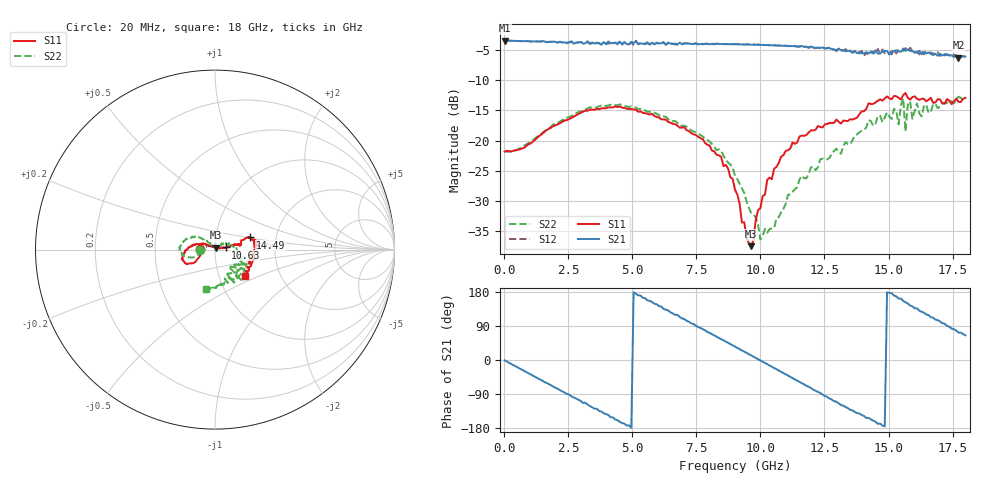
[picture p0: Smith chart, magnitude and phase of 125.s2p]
!Agilent Technologies,N5230A,US43500223,A.07.50.48
!Agilent N5230A: A.07.50.48
!Date: Monday, January 11, 2016 21:20:18
!Correction: S11(Full 2 Port(1,2))
!S21(Full 2 Port(1,2))
!S12(Full 2 Port(1,2))
!S22(Full 2 Port(1,2))
!S2P File: Measurements: S11, S21, S12, S22:
# Hz S  dB  R 50
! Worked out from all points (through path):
!   201 points, 20 MHz to 18 GHz, reference 50 ohm
!   highest |S21| = -3.44 dB at 20 MHz (marker M1); lowest = -6.3 dB at 17.73 GHz (marker M2)
!   group delay of S21, straight-line fit = 101 ps
!   lowest |S11| = -37.5 dB at 9.639 GHz (marker M3), VSWR 1.03, Z = 50.7 + j1.15 ohm
!   |S11| at or under -10 dB: start of sweep to end of sweep
!   |S22| runs from -36.4 to -12.7 dB; largest |S21 - S12| = 0.057
!   S11 on the Smith chart (normalised r, x): 20 MHz: 0.85, +0.00; 10.63 GHz: 1.13, +0.03; 14.49 GHz: 1.47, +0.21; 18 GHz: 1.33, -0.42
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2e7  -21.83 179.4  -3.44 -0.9  -3.43 -0.9  -21.76 180.0
1.5483e9  -18.66 -150.3  -3.54 -57.0  -3.57 -56.9  -18.55 -159.5
3.0766e9  -15.21 -153.1  -3.95 -113.3  -3.80 -112.2  -15.12 -168.7
4.515e9  -14.35 -165.2  -3.63 -163.2  -3.48 -162.3  -14.02 176.0
6.0433e9  -16.17 179.2  -3.92 142.1  -3.93 141.6  -15.78 157.3
7.4817e9  -19.07 163.7  -3.87 90.6  -4.00 90.9  -18.63 143.6
9.01e9  -28.14 149.7  -4.07 35.3  -4.02 35.6  -25.82 132.0
9.6393e9  -37.47 57.9  -4.14 12.2  -4.12 12.5  -31.96 114.4
9.9989e9  -31.19 10.7  -4.15 -1.3  -4.17 -0.8  -36.38 96.3
1.06282e10  -24.37 11.7  -4.28 -24.1  -4.25 -24.2  -32.86 51.4
1.20666e10  -18.33 13.7  -4.62 -78.4  -4.57 -77.7  -24.30 35.5
1.33252e10  -16.73 12.2  -5.22 -124.1  -4.85 -124.0  -20.26 14.3
1.44939e10  -13.71 19.2  -5.07 -163.0  -5.60 -159.7  -17.20 -13.3
1.50333e10  -13.02 12.5  -5.78 177.0  -5.43 175.9  -16.02 -33.4
1.53929e10  -12.94 8.2  -5.23 162.2  -5.00 167.0  -17.32 -38.4
1.55727e10  -12.49 5.4  -4.78 156.0  -5.18 161.2  -13.00 -49.1
1.56626e10  -12.12 5.0  -5.15 152.3  -4.68 153.2  -18.46 -51.1
1.58424e10  -13.22 4.3  -5.15 143.7  -4.63 145.3  -13.47 -60.3
1.59323e10  -12.79 1.2  -5.21 141.6  -5.14 139.7  -16.40 -63.2
1.6202e10  -13.26 -0.6  -5.14 130.2  -5.73 132.0  -15.49 -67.3
1.77303e10  -13.59 -36.0  -6.30 72.4  -5.87 74.5  -12.74 -99.2
1.8e10  -12.93 -41.6  -6.10 65.2  -6.16 64.2  -12.89 -103.3
